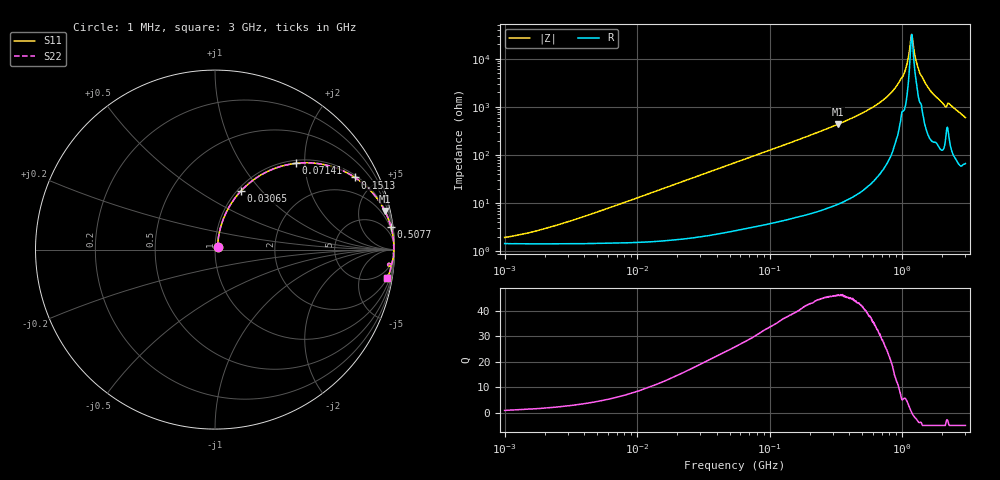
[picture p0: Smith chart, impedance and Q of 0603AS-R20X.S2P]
!s-Parameter Generated by FASTRON Sdn. Bhd.
!FASTRON P/N : 0603AS-R20X
!Keysight Technologies: E4991B_MY54100416_A.01.15
!Date created: Tue Oct 17 15:48:18 2023
!Version  : Rev01 Tue Oct 17 15:48:18 2023
!Data & Calibration Information:
!Freq	S11	S21	S12	S22
!PortZ  Port1:50+j0  Port2:50+j0
!When reading reference impedance value at option line is always used.
! Remarks : This data is being provided solely for informational purposes.
# Hz S dB R 50
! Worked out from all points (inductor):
!   1601 points, 1 MHz to 3 GHz, reference 50 ohm
!   read as one part in series: L = 205 nH near 3.374 MHz
!   highest Q = 45.9 at 326.9 MHz (marker M1), where L = 212 nH
!   self-resonance near 1.177 GHz
!   S11 on the Smith chart (normalised r, x): 1 MHz: 1.03, +0.03; 30.65 MHz: 1.04, +0.78; 71.41 MHz: 1.06, +1.80; 151.3 MHz: 1.10, +3.82; 507.7 MHz: 1, +15; 3 GHz: 2, -12
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1000000  -34.32 40.9  -0.13 -0.7  -0.13 -0.7  -34.32 40.9
3804036  -25.97 70.7  -0.14 -2.8  -0.14 -2.8  -25.97 70.7
1.447069e7  -14.91 74.7  -0.28 -10.3  -0.28 -10.3  -14.91 74.7
3.065274e7  -8.94 66.1  -0.76 -20.9  -0.76 -20.9  -8.94 66.1
5.477226e7  -5.05 53.8  -1.86 -34.0  -1.86 -34.0  -5.05 53.8
7.140691e7  -3.64 46.9  -2.72 -41.1  -2.72 -41.1  -3.64 46.9
1.512587e8  -1.14 27.3  -6.77 -61.2  -6.77 -61.2  -1.14 27.3
2.083556e8  -0.64 20.4  -9.15 -68.3  -9.15 -68.3  -0.64 20.4
3.268837e8  -0.26 12.8  -13.06 -75.9  -13.06 -75.9  -0.26 12.8
5.077325e8  -0.10 7.4  -17.76 -81.2  -17.76 -81.2  -0.10 7.4
7.925923e8  -0.04 3.2  -24.95 -84.2  -24.95 -84.2  -0.04 3.2
1.02815e9  -0.03 1.2  -33.52 -78.6  -33.52 -78.6  -0.03 1.2
1.086329e9  -0.02 0.7  -37.80 -76.8  -37.80 -76.8  -0.02 0.7
1.153559e9  -0.03 0.2  -46.68 -51.0  -46.68 -51.0  -0.03 0.2
1.182785e9  -0.03 -0.0  -50.12 1.8  -50.12 1.8  -0.03 -0.0
1.212752e9  -0.03 -0.2  -45.82 46.4  -45.82 46.4  -0.03 -0.2
1.274982e9  -0.04 -0.6  -39.06 66.5  -39.06 66.5  -0.04 -0.6
1.340405e9  -0.04 -1.0  -34.99 74.4  -34.99 74.4  -0.04 -1.0
1.596974e9  -0.04 -2.4  -27.50 81.9  -27.50 81.9  -0.04 -2.4
2.071593e9  -0.14 -5.1  -20.97 77.4  -20.97 77.4  -0.14 -5.1
2.289646e9  -0.15 -4.9  -21.22 76.0  -21.22 76.0  -0.15 -4.9
3e9  -0.27 -9.2  -15.83 74.4  -15.83 74.4  -0.27 -9.2
